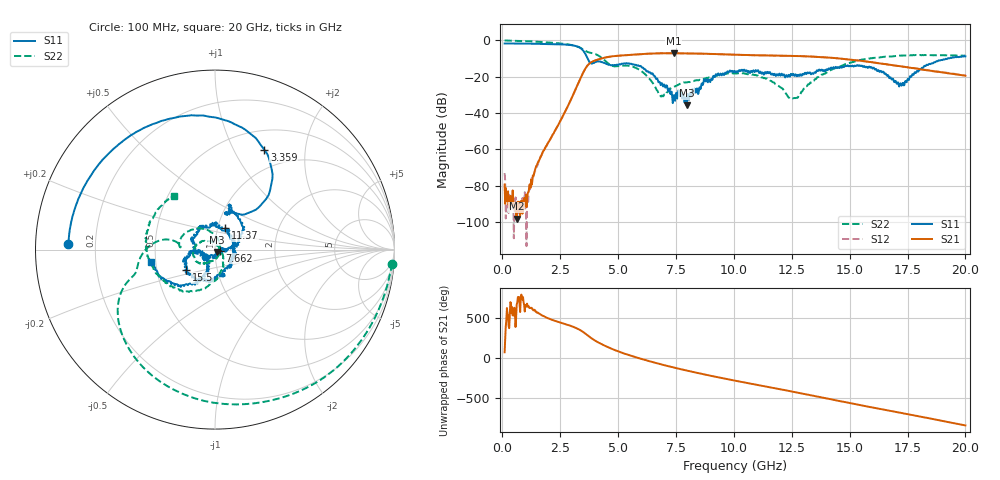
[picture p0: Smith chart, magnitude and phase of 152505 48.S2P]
!  2-Port S-parameters saved by WinCal
! VAR MeasName=S-Parameters (CALIBRATED_DATA) read from VNA (N5230C)
! VAR MeasDate=4/10/2015 9:33:20 AM
! VAR NAME=152505 48
! VAR FILENAME=152505 48.S2P
! VAR DATE=4/10/2015 9:33:20 AM
! VAR PHYS_PORTS=1,2
# Hz S DB R 50
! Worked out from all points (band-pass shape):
!   801 points, 100 MHz to 20 GHz, reference 50 ohm
!   highest |S21| = -7.11 dB at 7.413 GHz (marker M1); lowest = -98.0 dB at 622.4 MHz (marker M2)
!   |S21| within 3 dB of the highest: 4.25 GHz to 14.61 GHz (10.36 GHz wide, 110 % of centre)
!   lowest |S11| = -35.7 dB at 7.96 GHz (marker M3), VSWR 1.03, Z = 51 - j1.35 ohm
!   |S11| at or under -10 dB: 3.685 GHz to 19.24 GHz (15.55 GHz wide, 136 % of centre)
!   |S22| runs from -32.2 to -0.1 dB; largest |S21 - S12| = 0.0053
!   S11 on the Smith chart (normalised r, x): 100 MHz: 0.10, +0.02; 3.359 GHz: 0.73, +1.33; 7.662 GHz: 1.06, -0.01; 11.37 GHz: 1.09, +0.26; 15.5 GHz: 0.71, -0.17; 20 GHz: 0.47, -0.08
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1e8  -1.75 177.6  -79.30 71.3  -73.04 -79.8  -0.09 -4.5
6.22375e8  -1.78 165.1  -98.02 -47.3  -94.76 -27.6  -0.30 -25.3
1.1945e9  -1.86 151.1  -79.20 -93.3  -81.83 -88.3  -0.55 -48.3
2.33875e9  -2.14 118.0  -48.33 100.5  -48.30 99.7  -1.52 -96.2
3.358625e9  -4.14 63.8  -21.41 -8.8  -21.41 -8.5  -4.06 -149.8
3.43325e9  -4.87 57.4  -19.34 -21.9  -19.33 -21.7  -4.56 -153.9
4.303875e9  -12.01 68.4  -9.92 171.7  -9.91 171.6  -9.78 171.8
5.050125e9  -13.18 73.0  -8.42 78.2  -8.47 78.2  -14.13 175.8
5.871e9  -13.73 37.6  -7.73 0.3  -7.73 0.4  -15.81 134.8
6.741625e9  -23.02 4.9  -7.17 -70.4  -7.17 -70.6  -29.07 38.4
7.41325e9  -30.12 -8.4  -7.11 -119.6  -7.12 -119.6  -25.51 -86.1
7.662e9  -30.71 -11.9  -7.15 -137.0  -7.17 -136.8  -24.02 -101.6
7.9605e9  -35.74 -53.9  -7.21 -156.8  -7.18 -156.8  -23.13 -111.7
1.005e10  -16.95 146.0  -7.88 75.9  -7.93 75.7  -18.21 -158.0
1.136838e10  -17.55 64.3  -8.34 2.6  -8.32 2.7  -21.04 151.1
1.251262e10  -19.24 -9.9  -8.59 -61.1  -8.60 -60.8  -31.91 50.5
1.338325e10  -17.96 -56.8  -8.98 -110.8  -8.94 -110.6  -22.62 -53.4
1.549762e10  -14.15 -145.0  -11.25 126.7  -11.32 126.7  -10.73 -127.1
1.669162e10  -20.10 -171.4  -13.36 60.0  -13.38 59.6  -8.91 -162.2
1.723888e10  -24.95 -137.8  -14.37 30.0  -14.35 29.9  -8.39 -176.7
1.833338e10  -13.42 -117.9  -16.41 -30.0  -16.34 -30.8  -8.05 157.6
2e10  -8.83 -168.8  -19.46 -126.5  -19.41 -126.6  -8.48 127.8
